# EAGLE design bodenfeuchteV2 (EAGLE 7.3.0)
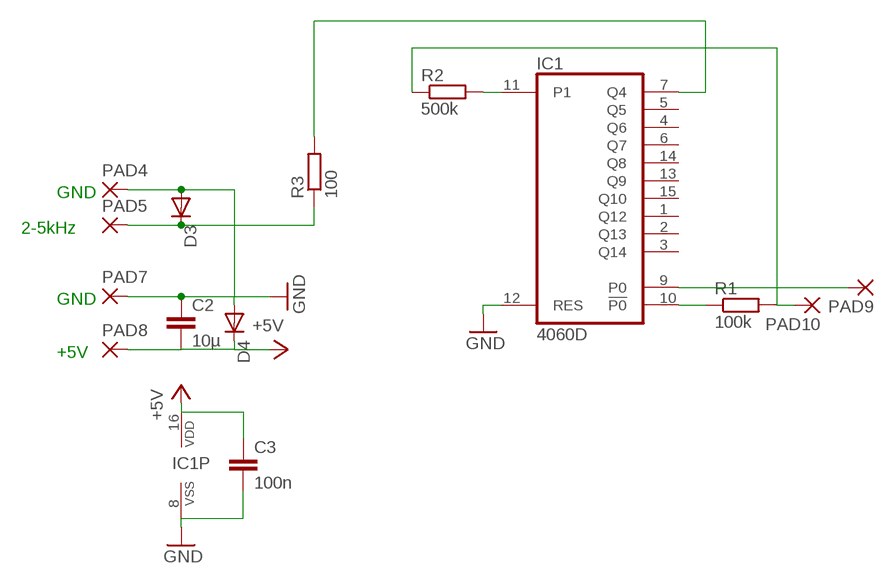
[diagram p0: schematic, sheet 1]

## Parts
C2  10µ  C-EUC1206  [C1206]
C3  100n  C-EUC0603  [C0603]
D3  DIODE-DO214AA  [DO214AA]
D4  DIODE-DO214AA  [DO214AA]
IC1  4060D  [SO16]
PAD4  2,15/1,0  [2,15/1,0]
PAD5  2,15/1,0  [2,15/1,0]
PAD7  2,15/1,0  [2,15/1,0]
PAD8  2,15/1,0  [2,15/1,0]
PAD9  2,15/1,0  [2,15/1,0]
PAD10  2,15/1,0  [2,15/1,0]
R1  100k  R-EU_R0603  [R0603]
R2  500k  R-EU_R0603  [R0603]
R3  100  R-EU_R1206  [R1206]

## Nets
+5V: C2.2 C3.1 D4.C IC1.16(VDD) PAD8.1(P)
GND: C2.1 C3.2 D3.A D4.A IC1.8(VSS) IC1.12(RES) PAD4.1(P) PAD7.1(P)
N$1: D3.C PAD5.1(P) R3.1
N$2: IC1.11(P1) R2.2
N$3: PAD10.1(P) R1.2 R2.1
N$4: IC1.10(!P0) R1.1
N$5: IC1.9(P0) PAD9.1(P)
N$6: IC1.7(Q4) R3.2
Unconnected: IC1.1(Q12) IC1.2(Q13) IC1.3(Q14) IC1.4(Q6) IC1.5(Q5) IC1.6(Q7) IC1.13(Q9) IC1.14(Q8) IC1.15(Q10)

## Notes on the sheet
- GND
- 2-5kHz
- GND
- +5V

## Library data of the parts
C2 C3 = rcl:C-EU: CAPACITOR, European symbol
D3 D4 = diode:DIODE-: DIODE
IC1 = 40xx:4060: 14-stage binary/ripple COUNTER
PAD4 PAD5 PAD7-PAD10 = wirepad:2,15/1,0: THROUGH-HOLE PAD
R1-R3 = rcl:R-EU_: RESISTOR, European symbol

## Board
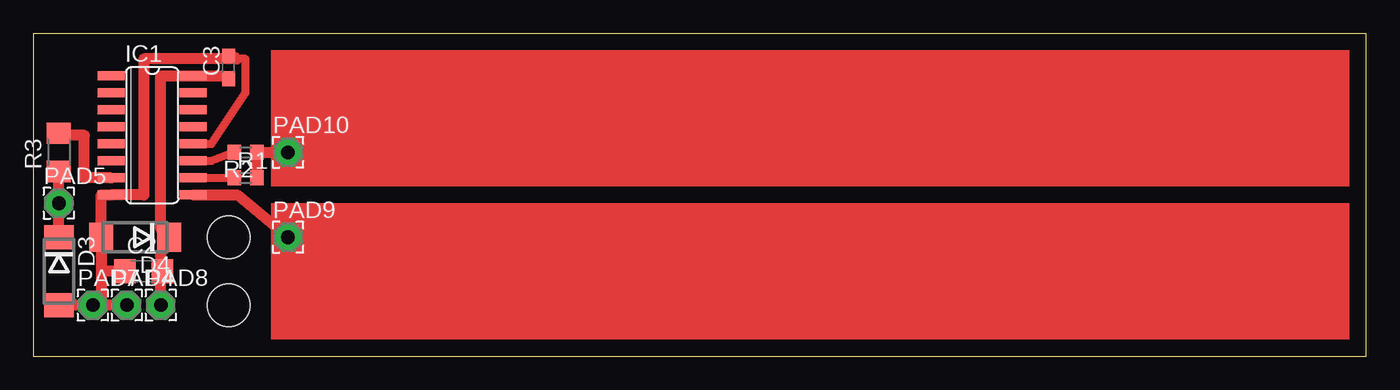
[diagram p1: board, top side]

Size 99.69 x 24.13 mm. Coordinates in mm from the lower left corner, seen from the top.
Outline: 96.83,24.12 0,24.12 0,0 99.69,0 99.69,24.13 96.52,24.13
Copper layers (1*16): Top 0.035mm / dielectric 1.5mm / Bottom 0.035mm
Design rules "default": minimum track width 10mil, minimum drill 24mil, track to track 8mil, track to pad 8mil, pad to pad 8mil, via to via 8mil, smd to smd 8mil, copper to edge 40mil, drill to drill 8mil, minimum pad ring 10mil, minimum via ring 8mil, stop-mask expansion 4mil, vias tented up to drill 0mil, thermal gap 10mil
Holes 3.2 mm at 14.61,3.81 14.61,8.89

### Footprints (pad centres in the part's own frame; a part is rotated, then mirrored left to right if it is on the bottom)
C1206 = smd 1.6 x 1.8: 1 -1.4,0; 2 1.4,0
C0603 = smd 1.1 x 1: 1 -0.85,0; 2 0.85,0
DO214AA = smd 1.8 x 2.2: A 2.55,0; C -2.55,0
SO16 = smd 0.66 x 2.032: 1 -4.445,-3.073; 2 -3.175,-3.073; 3 -1.905,-3.073; 4 -0.635,-3.073; 5 0.635,-3.073; 6 1.905,-3.073; 7 3.175,-3.073; 8 4.445,-3.073; 9 4.445,3.073; 10 3.175,3.073; 11 1.905,3.073; 12 0.635,3.073; 13 -0.635,3.073; 14 -1.905,3.073; 15 -3.175,3.073; 16 -4.445,3.073
2,15/1,0 = drill 1.016 pad 2.159 octagon: 1 0,0
R0603 = smd 1 x 1.1: 1 -0.85,0; 2 0.85,0
R1206 = smd 1.6 x 1.803: 1 -1.422,0; 2 1.422,0

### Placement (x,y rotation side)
C2  8.26,6.35 0 top
C3  14.61,21.59 90 top
D3  1.91,6.35 270 top
D4  7.62,8.89 180 top
IC1  8.89,16.51 270 top
PAD4  6.99,3.81 0 top
PAD5  1.91,11.43 0 top
PAD7  4.45,3.81 0 top
PAD8  9.53,3.81 0 top
PAD9  19.05,8.89 0 top
PAD10  19.05,15.24 0 top
R1  15.88,13.34 0 top
R2  15.88,15.24 180 top
R3  1.91,15.24 90 top

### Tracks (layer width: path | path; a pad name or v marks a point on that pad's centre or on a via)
+5V
  Top 0.813: C3.1 13.97,20.95 IC1.16 9.53,20.95 9.53,9.53 D4.C 9.53,7.62 C2.2 9.53,5.71 PAD8.1
GND
  Top 0.61: IC1.12 13.34,15.88 15.88,19.68 15.88,22.23 15.24,22.23
  Top 0.813: C3.2 15.24,22.23 8.26,22.23 8.26,12.06 IC1.8 5.08,12.06 D4.A 5.08,9.53 5.08,6.35 | PAD7.1 D3.A | 5.08,6.35 5.08,3.81 PAD7.1 | PAD4.1 PAD7.1 | C2.1 5.08,6.35
N$1
  Top 0.813: R3.1 PAD5.1 D3.C
N$2
  Top 0.61: IC1.11 13.34,14.61 R2.2
N$3
  Top 0.813: R1.2 R2.1 PAD10.1
N$4
  Top 0.61: IC1.10 R1.1
N$5
  Top 0.813: IC1.9 15.24,12.06 PAD9.1
N$6
  Top 0.813: IC1.7 3.81,13.34 3.81,16.51 1.91,16.51 R3.2
(copper drawn outside any net)
  shapes: Top area x6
